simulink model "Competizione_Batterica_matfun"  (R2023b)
settings: Solver=ode45  StartTime=0.0  StopTime=10  RelTol=1e-6  EnableMultiTasking=on

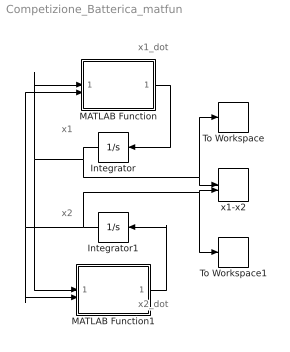
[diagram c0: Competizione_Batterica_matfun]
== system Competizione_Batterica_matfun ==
  note: x1_dot
  note: x2_dot
  note: x2
  note: x1
  Integrator : Integrator  InitialCondition=0.5
  Integrator1 : Integrator  InitialCondition=2
  MATLAB Function : MATLAB Function  TreatAsAtomicUnit=on
  MATLAB Function1 : MATLAB Function  TreatAsAtomicUnit=on
  To Workspace : ToWorkspace  VariableName=x1  SampleTime=-1
  To Workspace1 : ToWorkspace  VariableName=x2  SampleTime=-1
  x1-x2 : Record  FileSettingsInternal="{\"entries\":[{\"content\":{\"excelSettings\":{\"content\":{},\"type\":\"Streamout.ExcelSettings\"}},\"type\":\"Streamout.FileSettingStorage\",\"uuid\":\"\"}],\"packageUris\":[\"http:\\/\\/schema.mathworks.com\\/mf0\\/streamout_blocks\\/R2020a\"],\"version\":\"1.0\"}"  Layout=[1 1]  SignalsInternal="{\"entries\":[{\"content\":{\"signals\":[{\"content\":{\"blockPath\":[],\"dimensions\":[1],\"domain\":\"\",\"lineColor\":\"#a2142f\",\"plots\":[ 1 ],\"port\":1,\"sid\":[\"\"],\"signalID\":1,\"signalName\":\"Integrator\"},\"type\":\"RecordBlkView.Signal\",\"uuid\":\"\"},{\"content\":{\"blockPath\":[],\"dimensions\":[1],\"domain\":\"\",\"lineColor\":\"#139fff\",\"plots\":[ 1 ],\"port\":2,\"sid\":[\"\"],\"signalID\":2,\"signalName\":\"Integrator1\"},\"type\":\"RecordBlkVi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"  VisualizationBindings="{\"xyplotplugin\":{\"info\":[{\"series\":[{\"bindingParametersList\":[{\"parameter\":\"X-Axis\",\"signalID\":1,\"signalName\":\"Integrator\"},{\"parameter\":\"Y-Axis\",\"signalID\":2,\"signalName\":\"Integrator1\"}],\"seriesID\":0}],\"subplotID\":1}]}}"  CompatibilityTag=XY  st=0.01
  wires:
  MATLAB Function/1(y) -> Integrator/1
  MATLAB Function1/1(y) -> Integrator1/1
  Integrator/1 -> MATLAB Function/1(x1), MATLAB Function1/1(x1), To Workspace/1, x1-x2/1
  Integrator1/1 -> MATLAB Function/2(x2), MATLAB Function1/2(x2), To Workspace1/1, x1-x2/2

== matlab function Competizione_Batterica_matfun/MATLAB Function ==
function y = fcn_x1_dot(x1,x2)

y = 5*x1*(1-x1/1)-10*x1*x2;

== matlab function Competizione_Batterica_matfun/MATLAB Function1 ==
function y = fcn_x2_dot(x1,x2)

y = 5*x2*(1-x2/2)-10*x1*x2;
